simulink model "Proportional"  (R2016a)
settings: Solver=VariableStepAuto  StartTime=0.0  StopTime=10.0  RelTol=1e-3
libraries: vexarmcortexlib x6

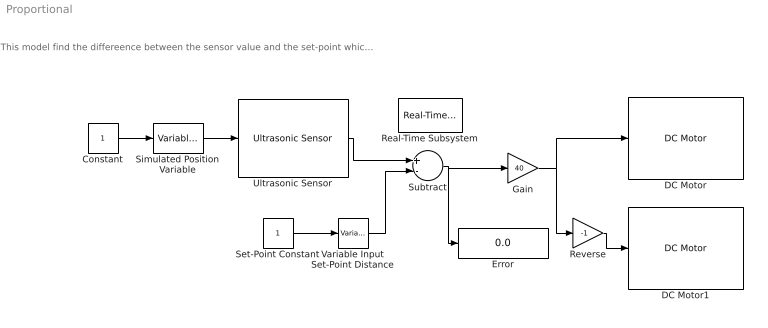
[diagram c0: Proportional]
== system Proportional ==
  note: This model find the differeence between the sensor value and the set-point which we call the error. The error is multiplied by the gain to control the speed of the motors.
  Constant : Constant
  DC Motor : vexarmcortexlib/DC Motor  motor=3  scaleFactor=1/13.5  SimulationOut=on
  DC Motor1 : vexarmcortexlib/DC Motor  motor=7  scaleFactor=1/13.5  SimulationOut=on
  Error : Display
  Gain : Gain  Gain=40
  Real-Time Subsystem : vexarmcortexlib/Utilities/Real-Time Subsystem  x=1
  Reverse : Gain  Gain=-1
  Set-Point Constant : Constant
  Simulated Position Variable : vexarmcortexlib/Utilities/Variable Input  low=0  gain=2  high=2
  Subtract : Sum  Inputs=+-
  Ultrasonic Sensor : vexarmcortexlib/Ultrasonic Sensor  inputPin=3  outputPin=2  inputPortSim=on  SampleTime=0.2
  Variable Input Set-Point Distance : vexarmcortexlib/Utilities/Variable Input  low=0  gain=0.2  high=2
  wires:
  Ultrasonic Sensor/1 -> Subtract/1
  Subtract/1 -> Error/1, Gain/1
  Gain/1 -> DC Motor/1, Reverse/1
  Reverse/1 -> DC Motor1/1
  Variable Input Set-Point Distance/1 -> Subtract/2
  Set-Point Constant/1 -> Variable Input Set-Point Distance/1
  Simulated Position Variable/1 -> Ultrasonic Sensor/1
  Constant/1 -> Simulated Position Variable/1
